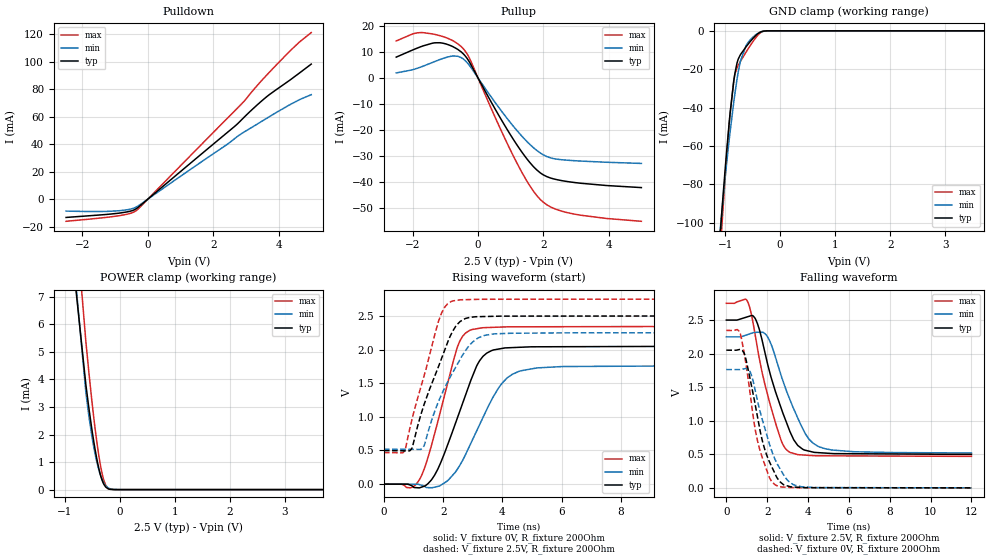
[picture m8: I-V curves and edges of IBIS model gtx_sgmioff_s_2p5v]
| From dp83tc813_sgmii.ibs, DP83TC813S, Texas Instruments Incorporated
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| gtx_sgmioff_s_2p5v
[Model]   gtx_sgmioff_s_2p5v
Model_type   I/O
Polarity   Non-Inverting
Enable   Active-Low
Vinl = 0.7
Vinh = 1.7
Vmeas = 1.25
Vref = 1.25
Cref = 2pF
Rref = 100000
|   typ   min   max
C_comp   4.12pF   3.94pF   4.21pF
[Voltage Range]   2.5   2.25   2.75
[Temperature Range]   27   150   -40
[Pullup Reference]   2.5   2.25   2.75
[Pulldown Reference]   -0   -0   0
[Power Clamp Reference]   2.5   2.25   2.75
[GND Clamp Reference]   0   0   0
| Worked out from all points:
|   slope of the pulldown table from 0 to 0.375 V, typ, clamps not added: 49.7 ohm
|   slope of the pullup table from 0 to 0.375 V, typ, clamps not added: 43.5 ohm
|   GND clamp passes 1 mA (typ) near -0.38 V on its own axis
|   POWER clamp passes 1 mA (typ) near -0.41 V on its own axis
|   falling waveform, V_fixture 2.5V, R_fixture 200Ohm: 20-80 % time 1.21ns typ, 1.32ns min, 1.04ns max; typ from 2.5 V to 0.498 V
|   rising waveform, V_fixture 0V, R_fixture 200Ohm: 20-80 % time 1.02ns typ, 1.18ns min, 837ps max; typ from 0 V to 2.05 V
|   rising waveform, V_fixture 2.5V, R_fixture 200Ohm: 20-80 % time 982ps typ, 1.08ns min, 833ps max; typ from 0.498 V to 2.5 V
|   falling waveform, V_fixture 0V, R_fixture 200Ohm: 20-80 % time 924ps typ, 1.05ns min, 795ps max; typ from 2.05 V to 0 V
[Pulldown]
|   Voltage   I(typ)   I(min)   I(max)
-2.5V     -13.29mA   -8.687mA   -16.1mA
-925mV    -10.31mA   -8.492mA   -12.22mA
-512.5mV  -8.603mA   -7.139mA   -10.18mA
-347.5mV  -6.835mA   -5.631mA   -8.211mA
2.638V    52.57mA    43.69mA    63.75mA
2.885V    58.13mA    47.96mA    69.7mA
3.462V    71.02mA    56.29mA    85.76mA
3.958V    80.11mA    63.41mA    98.27mA
4.633V    91.66mA    72.28mA    114.2mA
5V        98.27mA    76.01mA    121.2mA
[GND Clamp]
|   Voltage   I(typ)   I(min)   I(max)
-2.5V     -712.2mA   -617mA     -795.7mA
-1.105V   -112.1mA   -109mA     -122.5mA
-1.045V   -89.14mA   -90.27mA   -96.16mA
-970mV    -62.33mA   -68.65mA   -65.01mA
-910mV    -43.44mA   -53.04mA   -43.24mA
-842.5mV  -26.37mA   -37.26mA   -25.92mA
-782.5mV  -16.71mA   -25.15mA   -19.21mA
-722.5mV  -12.49mA   -15.9mA    -16.01mA
-617.5mV  -8.274mA   -7.642mA   -11.03mA
-497.5mV  -4.092mA   -3.395mA   -5.748mA
-355mV    -617.9uA   -659.9uA   -973.5uA
5V        0A         0A         0A
[Pullup]
|   Voltage   I(typ)   I(min)   I(max)
-2.5V     7.944mA    1.866mA    14.16mA
-1.847V   11.46mA    3.684mA    17.29mA
-1.315V   13.45mA    6.279mA    16.67mA
-752.5mV  11.89mA    8.383mA    14.16mA
-460mV    9.358mA    7.341mA    11.34mA
-257.5mV  5.988mA    4.704mA    7.488mA
642.5mV   -14.55mA   -11.48mA   -18.41mA
1.272V    -27.27mA   -21.43mA   -34.67mA
1.677V    -33.87mA   -26.64mA   -43.23mA
2.007V    -37.38mA   -29.68mA   -47.92mA
2.953V    -40.27mA   -31.88mA   -52.42mA
5V        -42.22mA   -32.93mA   -55.18mA
[POWER Clamp]
|   Voltage   I(typ)   I(min)   I(max)
-2.5V     111.4mA    76.19mA    154.9mA
-1.06V    12.26mA    13.09mA    16.05mA
-617.5mV  3.803mA    3.522mA    5.367mA
-557.5mV  2.879mA    2.591mA    4.147mA
-505mV    2.141mA    1.896mA    3.157mA
-445mV    1.398mA    1.242mA    2.137mA
-392.5mV  857.5uA    791.9uA    1.369mA
-347.5mV  495.5uA    495.6uA    828.3uA
-302.5mV  241.6uA    280.6uA    419.5uA
-220mV    36.62uA    73.16uA    55.78uA
-2.5mV    0A         192.6nA    0A
5V        0A         0A         0A
[Ramp]
R_load = 200
|   typ   min   max
dV/dt_r   1.23034/1.01648e-09   1.05661/1.18366e-09   1.40714/8.34439e-10
dV/dt_f   1.20094/1.2083e-09   1.03795/1.31409e-09   1.36847/1.04384e-09
[Falling Waveform]
V_fixture = 2.5V
V_fixture_min = 2.25V
V_fixture_max = 2.75V
R_fixture = 200Ohm
C_fixture = 0F
|   Time   V(typ)   V(min)   V(max)
0s        2.5V       2.25V      2.75V
1.062ns   2.551V     2.286V     2.763V
1.448ns   2.503V     2.317V     2.216V
1.991ns   1.883V     2.264V     1.421V
2.687ns   1.185V     1.669V     702.5mV
3.067ns   875.6mV    1.349V     537.7mV
3.496ns   632.2mV    1.041V     495.5mV
4.031ns   548.4mV    731.8mV    484.5mV
4.831ns   518.4mV    583.2mV    477.4mV
12ns      498.4mV    520mV      469.2mV
[Rising Waveform]
V_fixture = 0V
V_fixture_min = 0V
V_fixture_max = 0V
R_fixture = 200Ohm
C_fixture = 0F
|   Time   V(typ)   V(min)   V(max)
0s        26.53uV    136.2uV    12.21uV
889.1ps   -14.84mV   -736.9uV   -55.44mV
1.216ns   -53.09mV   -9.637mV   81.87mV
1.711ns   134.1mV    -45.28mV   751.8mV
2.461ns   963.6mV    211.2mV    2.014V
2.887ns   1.488V     564.6mV    2.284V
3.469ns   1.947V     1.109V     2.327V
3.995ns   2.018V     1.505V     2.335V
4.621ns   2.035V     1.685V     2.339V
12ns      2.051V     1.761V     2.345V
[Rising Waveform]
V_fixture = 2.5V
V_fixture_min = 2.25V
V_fixture_max = 2.75V
R_fixture = 200Ohm
C_fixture = 0F
|   Time   V(typ)   V(min)   V(max)
0s        498.4mV    520mV      469.2mV
707.1ps   495mV      517.6mV    499.8mV
942ps     531.3mV    516.8mV    952.9mV
1.35ns    1.178V     566.5mV    1.605V
1.861ns   1.771V     1.249V     2.446V
2.26ns    2.221V     1.611V     2.713V
2.572ns   2.418V     1.856V     2.74V
2.972ns   2.482V     2.104V     2.745V
3.718ns   2.495V     2.234V     2.748V
12ns      2.5V       2.25V      2.75V
[Falling Waveform]
|Gnd
V_fixture = 0V
V_fixture_min = 0V
V_fixture_max = 0V
R_fixture = 200Ohm
C_fixture = 0F
|   Time   V(typ)   V(min)   V(max)
0s        2.052V     1.762V     2.346V
613.4ps   2.059V     1.762V     2.339V
881.4ps   2V         1.775V     1.991V
1.164ns   1.622V     1.73V      1.405V
1.522ns   1.063V     1.304V     707.1mV
1.875ns   580.2mV    897.6mV    351.2mV
2.383ns   211.1mV    424.7mV    46.57mV
3.016ns   27.12mV    105.4mV    8.094mV
3.698ns   5.612mV    15.28mV    2.316mV
12ns      26.61uV    136.4uV    12.33uV
